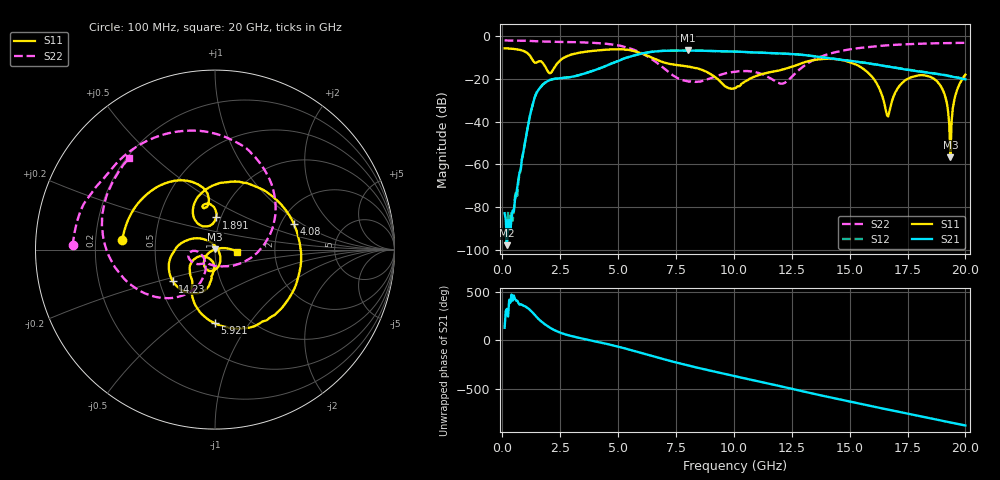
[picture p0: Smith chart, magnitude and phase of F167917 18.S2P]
!  2-Port S-parameters saved by WinCal
! VAR MeasName=S-Parameters (CALIBRATED_DATA) read from VNA (N5242A)
! VAR MeasDate=2016-11-22 9:00:37
! VAR NAME=F167917 18
! VAR FILENAME=F167917 18.S2P
! VAR DATE=2016-11-22 9:00:37
! VAR PHYS_PORTS=1,2
# Hz S DB R 50
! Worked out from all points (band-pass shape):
!   401 points, 100 MHz to 20 GHz, reference 50 ohm
!   highest |S21| = -6.72 dB at 8.01 GHz (marker M1); lowest = -97.8 dB at 199.5 MHz (marker M2)
!   |S21| within 3 dB of the highest: 5.468 GHz to 13.68 GHz (8.214 GHz wide, 85.8 % of centre)
!   lowest |S11| = -56.7 dB at 19.35 GHz (marker M3), VSWR 1.00, Z = 50.1 + j0.118 ohm
!   |S11| at or under -10 dB: 1.246 GHz to 2.676 GHz (1.43 GHz wide, 73 % of centre); 6.447 GHz to end of sweep
!   |S22| runs from -22.2 to -2.0 dB; largest |S21 - S12| = 0.004
!   S11 on the Smith chart (normalised r, x): 100 MHz: 0.32, +0.05; 1.891 GHz: 0.95, +0.35; 4.08 GHz: 2.34, +0.86; 5.921 GHz: 0.71, -0.70; 14.23 GHz: 0.59, -0.23; 20 GHz: 1.29, -0.03
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1e8  -5.71 174.2  -82.79 129.7  -93.98 -66.5  -2.03 178.3
1.995e8  -5.75 168.3  -97.80 -34.7  -98.18 19.7  -2.04 176.7
5.4775e8  -6.05 147.4  -76.47 67.2  -74.98 88.3  -2.09 171.0
1.3935e9  -12.33 100.6  -28.79 -95.1  -28.78 -95.3  -2.36 157.2
1.891e9  -14.93 88.1  -21.49 157.0  -21.46 156.8  -2.59 149.8
3.43325e9  -7.59 57.8  -17.87 18.6  -17.87 18.5  -2.91 122.9
4.08e9  -6.72 18.3  -15.56 -14.8  -15.56 -14.9  -3.23 107.3
5.92075e9  -7.75 -90.4  -8.41 -124.9  -8.36 -124.9  -7.45 37.4
6.7665e9  -11.46 -119.3  -7.00 178.0  -6.98 177.9  -13.19 -8.8
8.01025e9  -14.23 -135.3  -6.72 101.9  -6.68 101.8  -21.10 -97.4
1.005e10  -24.34 -113.3  -7.25 -10.4  -7.25 -10.3  -16.70 -154.3
1.208975e10  -15.65 -96.8  -8.16 -118.1  -8.10 -118.2  -22.20 -146.0
1.338325e10  -11.35 -115.5  -9.29 171.2  -9.25 171.5  -11.48 -119.7
1.4229e10  -10.62 -142.9  -10.49 127.4  -10.44 127.5  -7.93 -137.8
1.577125e10  -16.82 155.5  -12.68 48.7  -12.68 49.2  -5.13 -167.4
1.67165e10  -35.34 -6.2  -14.29 1.5  -14.31 2.2  -4.24 177.5
1.726375e10  -21.92 -70.4  -15.33 -25.3  -15.24 -24.3  -3.88 169.3
1.83085e10  -18.50 -113.7  -17.02 -75.2  -16.84 -75.2  -3.44 154.4
1.9005e10  -24.70 -145.9  -18.06 -110.0  -17.95 -110.1  -3.30 145.3
1.935325e10  -56.65 53.5  -18.81 -127.9  -18.65 -127.8  -3.22 141.1
1.9602e10  -26.53 9.9  -19.28 -140.3  -19.21 -140.1  -3.17 138.0
2e10  -18.00 -5.7  -20.17 -159.0  -20.05 -158.7  -3.12 133.0
